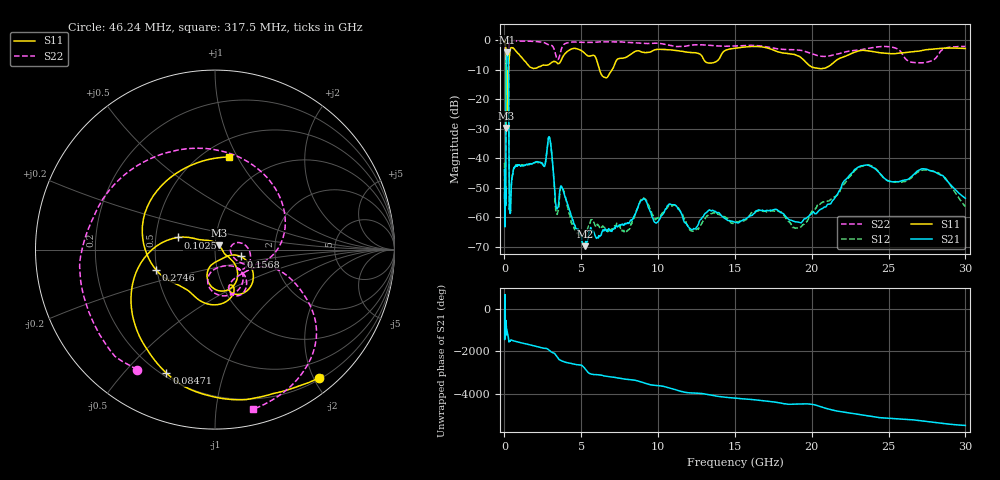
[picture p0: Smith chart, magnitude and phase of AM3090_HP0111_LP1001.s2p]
! Date/Time: Thu, Feb 28, 2019 2:01 PM
! Network Analyzer: Agilent Technologies E8364B Rev: A.07.50.67
! Sweep from 0.010 to 30.000 GHz, 1601 Points, Sweep Type: LOG
! Power Supply: 5.023 V, 0.002 A
# Hz S DB R 50
!freq MagS11 AngS11 MagS21 AngS21 MagS12 AngS12 MagS22 AngS22
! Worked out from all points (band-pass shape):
!   1601 points, 10 MHz to 30 GHz, reference 50 ohm
!   highest |S21| = -4.13 dB at 162.4 MHz (marker M1); lowest = -69.9 dB at 5.232 GHz (marker M2)
!   |S21| within 3 dB of the highest: 114.2 MHz to 250.4 MHz (136.2 MHz wide, 74.7 % of centre)
!   lowest |S11| = -29.8 dB at 109.9 MHz (marker M3), VSWR 1.07, Z = 52.2 + j2.43 ohm
!   |S11| at or under -10 dB: 100.6 MHz to 269.6 MHz (169 MHz wide, 91.3 % of centre); 6.184 GHz to 7.011 GHz (826.3 MHz wide, 12.5 % of centre)
!   |S22| runs from -21.4 to -0.1 dB; largest |S21 - S12| = 0.013
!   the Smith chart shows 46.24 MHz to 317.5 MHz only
!   S11 on the Smith chart (normalised r, x): 46.24 MHz: 0.22, -2.08; 84.71 MHz: 0.22, -0.66; 102.5 MHz: 0.65, +0.09; 156.8 MHz: 1.33, -0.10; 274.6 MHz: 0.50, -0.13; 317.5 MHz: 0.65, +0.93
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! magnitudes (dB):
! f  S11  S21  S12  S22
! 10 MHz  -0.2  -44.2  -41.9  -0.6
! 38.04 MHz  -0.5  -60.6  -60.4  -1.5
! 46.24 MHz  -0.7  -51.7  -53.6  -2.0
! 84.71 MHz  -2.6  -53.6  -49.6  -4.8
! 102.5 MHz  -13.3  -16.5  -16.4  -11.7
! 109.9 MHz  -29.8  -8.8  -8.8  -20.9
! 125.2 MHz  -12.7  -5.6  -5.5  -14.7
! 144.7 MHz  -23.6  -4.4  -4.4  -15.4
! 156.8 MHz  -16.6  -4.2  -4.1  -14.8
! 162.4 MHz  -13.4  -4.1  -4.1  -13.5
! 274.6 MHz  -9.2  -17.7  -17.7  -7.3
! 317.5 MHz  -5.6  -56.2  -57.2  -0.8
! 550.5 MHz  -2.7  -45.0  -44.6  -0.2
! 2.084 GHz  -9.5  -41.2  -41.3  -0.5
! 2.928 GHz  -8.2  -32.9  -33.0  -1.6
! 3.402 GHz  -7.6  -57.2  -59.0  -6.3
! 5.232 GHz  -4.5  -69.9  -66.5  -0.8
! 7.926 GHz  -5.8  -62.3  -64.9  -0.8
! 9.027 GHz  -4.1  -53.8  -53.4  -1.1
! 19.12 GHz  -5.4  -61.7  -63.7  -3.4
! 23.48 GHz  -3.5  -42.4  -42.4  -3.0
! 30 GHz  -2.9  -53.6  -56.5  -2.2
